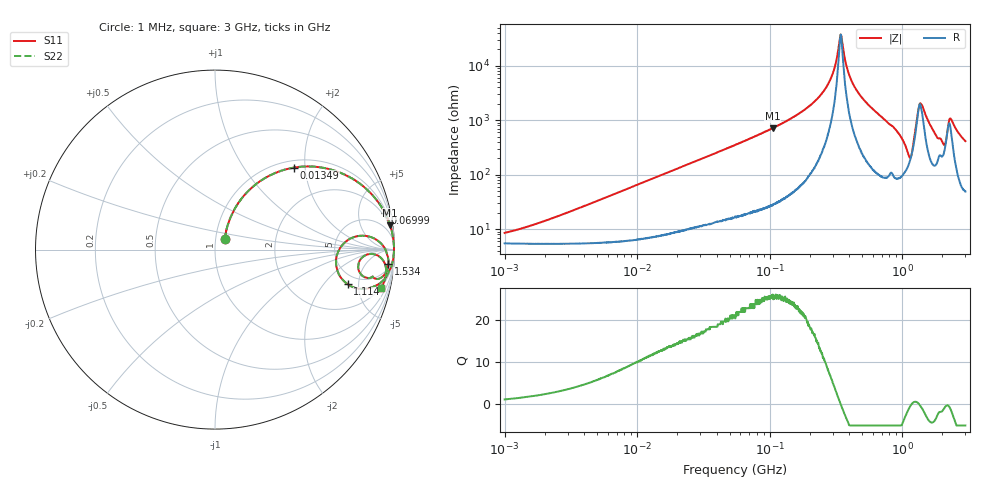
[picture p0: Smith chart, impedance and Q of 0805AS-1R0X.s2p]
!s-Parameter Generated by FASTRON Sdn. Bhd.
!FASTRON P/N : 0805AS-1R0X
!Keysight Technologies: E4991B_MY54100416_A.01.15
!Date: Mon Jun 15 12:56:32 2026
!Version  :Rev01  Mon Jun 15 12:56:32 2026
!Data & Calibration Information:
!Freq  S11  S21  S12  S22
!PortZ  Port1:50+j0  Port2:50+j0
!When reading reference impedance value at option line is always used.
! Remarks : This data is being provided solely for informational purposes.
# Hz S dB R 50
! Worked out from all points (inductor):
!   1601 points, 1 MHz to 3 GHz, reference 50 ohm
!   read as one part in series: L = 1.04 uH near 2.474 MHz
!   highest Q = 25.7 at 105.5 MHz (marker M1), where L = 1.08 uH
!   self-resonance near 343.7 MHz
!   S11 on the Smith chart (normalised r, x): 1 MHz: 1.11, +0.13; 13.49 MHz: 1.14, +1.74; 69.99 MHz: 1.40, +9.07; 1.114 GHz: 3.96, -3.66; 1.534 GHz: 8, -21; 3 GHz: 1.98, -8.24
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1000000  -21.90 46.4  -0.48 -3.5  -0.48 -3.5  -21.90 46.4
3804036  -12.60 64.4  -0.69 -13.2  -0.69 -13.2  -12.60 64.4
1.349163e7  -3.98 46.2  -2.80 -39.1  -2.80 -39.1  -3.98 46.2
1.447069e7  -3.64 44.5  -3.06 -41.0  -3.06 -41.0  -3.64 44.5
5.504702e7  -0.44 15.6  -11.40 -71.6  -11.40 -71.6  -0.44 15.6
6.999185e7  -0.29 12.3  -13.40 -75.2  -13.40 -75.2  -0.29 12.3
1.054994e8  -0.13 7.9  -17.20 -79.9  -17.20 -79.9  -0.13 7.9
2.083556e8  -0.04 2.9  -26.00 -83.9  -26.00 -83.9  -0.04 2.9
2.841474e8  -0.02 1.1  -34.50 -81.0  -34.50 -81.0  -0.02 1.1
3.453811e8  -0.02 -0.0  -51.20 8.0  -51.20 8.0  -0.02 -0.0
3.894533e8  -0.03 -0.7  -38.10 75.7  -38.10 75.7  -0.03 -0.7
4.435663e8  -0.03 -1.5  -31.80 81.3  -31.80 81.3  -0.03 -1.5
7.925923e8  -0.16 -6.5  -18.90 77.3  -18.90 77.3  -0.16 -6.5
9.878038e8  -0.51 -11.2  -14.10 67.7  -14.10 67.7  -0.51 -11.2
1.113852e9  -2.34 -14.6  -9.77 36.5  -9.77 36.5  -2.34 -14.6
1.188719e9  -2.77 3.3  -11.10 -8.7  -11.10 -8.7  -2.77 3.3
1.360679e9  -0.41 -0.5  -26.50 10.5  -26.50 10.5  -0.41 -0.5
1.534307e9  -0.27 -4.8  -21.20 67.3  -21.20 67.3  -0.27 -4.8
1.791767e9  -0.56 -9.7  -15.20 64.2  -15.20 64.2  -0.56 -9.7
2.03054e9  -1.40 -10.5  -13.00 43.4  -13.00 43.4  -1.40 -10.5
2.324278e9  -0.53 -3.9  -21.10 46.4  -21.10 46.4  -0.53 -3.9
3e9  -0.47 -13.1  -12.80 70.1  -12.80 70.1  -0.47 -13.1
